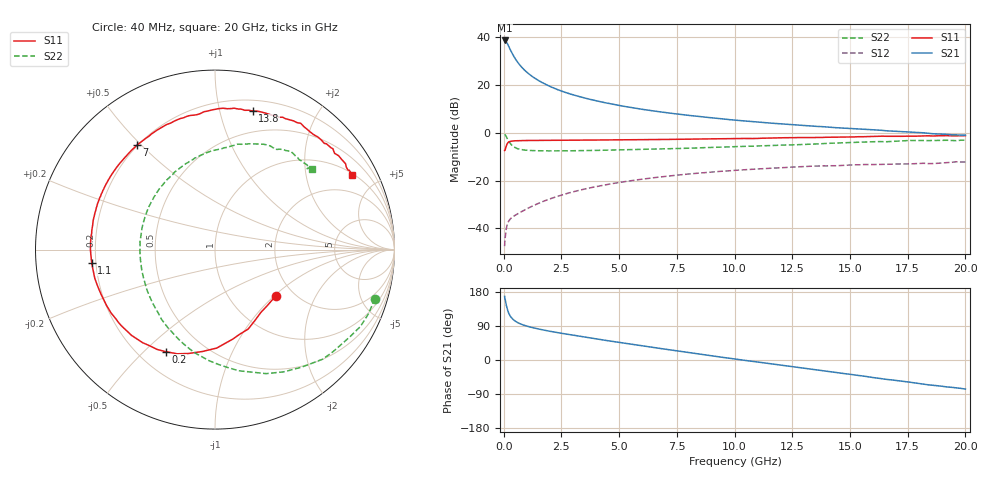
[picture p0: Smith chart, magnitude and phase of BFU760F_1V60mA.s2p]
! Filename:  P:\Prog\Test\Noise\ATS_data\Testdata_Net\Split files Spar\BFU760F_2W_C1_1V_5mA_60mA_Bias9_D.s2p
! Date/Time: Mon 06/Feb/2012 15:06:24
! BFU760_2W_C1_1V_5mA_60mA_Bias9_R.s2p
! MDIF S-parameter v. bias file
! BFU760_2W_C1_1V_5mA_60mA
! Date/time Fri Mar 18 10:56:44 2011
! VAR V_out= 1.0003
! VAR I_out= 60.0200
! VAR V_in= 0.8205
! VAR I_in= 0.2130
! Device data file deembeded for feedlines and parallel
! Original file: \Split files Spar\BFU760_2W_C1_1V_5mA_60mA_Bias9_R.s2p
! Feed-files: PR003V01_101208_Feed1.s2p, PR003V01_101208_Feed2.s2p
! Parallel-file: PR003V01_101208_Par.s2p
# MHz S MA R 50
!  Freq-MHz  S11-mag  S11-arg  S21-mag  S21-arg  S12-mag  S12-arg  S22-mag  S22-arg
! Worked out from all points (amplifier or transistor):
!   167 points, 40 MHz to 20 GHz, reference 50 ohm
!   highest |S21| = 38.7 dB at 40 MHz (marker M1)
!   |S21| within 3 dB of that: start of sweep to 241.6 MHz
!   unconditionally stable (mu >= 1): 2.694 GHz to 15.28 GHz
!   at 550 MHz: K = 0.55, MSG = 32.3 dB, |S12| = -34.3 dB
!   at 4.2 GHz: K = 1.04, MAG = 16.4 dB, |S12| = -22.2 dB
!   at 20 GHz: K = 0.96, MSG = 5.6 dB, |S12| = -12.3 dB
!   S11 on the Smith chart (normalised r, x): 40 MHz: 1.63, -1.02; 200 MHz: 0.31, -0.58; 1.1 GHz: 0.18, -0.05; 7 GHz: 0.20, +0.48; 13.8 GHz: 0.30, +1.26; 20 GHz: 1.06, +3.65
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40  0.4258 -37.1  86.21 167.8  0.004202 78.3  0.9318 -17.1
50  0.4273 -47.5  84.01 162.9  0.005292 70.9  0.9271 -22.6
60  0.4336 -54.0  79.17 160.6  0.005886 71.9  0.9167 -27.8
80  0.48 -67.4  82.28 154.5  0.007572 68.0  0.8807 -36.7
120  0.5486 -89.0  78.46 142.8  0.01019 60.3  0.813 -53.8
180  0.6175 -109.9  71.24 129.7  0.01293 52.3  0.7128 -73.3
200  0.6312 -115.7  67.27 126.2  0.01359 50.4  0.6879 -78.9
260  0.6569 -127.9  58.51 118.2  0.01508 46.7  0.6196 -93.1
300  0.6669 -134.3  53.08 114.3  0.01586 45.2  0.5869 -100.8
380  0.6739 -143.4  45.04 108.6  0.0171 43.6  0.5327 -113.6
480  0.6792 -151.6  37.07 103.3  0.01844 43.5  0.4952 -125.4
750  0.6864 -164.5  24.64 94.7  0.02198 46.2  0.4463 -145.4
1100  0.6906 -174.0  17.02 87.8  0.02693 50.2  0.4271 -159.8
2000  0.6933 172.2  9.4 75.8  0.0411 54.0  0.4186 -179.1
3400  0.7026 157.8  5.532 61.6  0.06442 51.0  0.424 163.8
6800  0.7241 128.4  2.738 30.3  0.1189 32.4  0.4586 132.5
7000  0.7266 126.8  2.656 28.6  0.1218 31.2  0.4623 130.8
10200  0.7592 101.8  1.811 1.1  0.1651 9.9  0.5147 105.4
13400  0.7937 77.9  1.379 -24.9  0.2 -12.6  0.5797 82.0
13800  0.7995 74.8  1.346 -28.2  0.2027 -15.5  0.592 79.2
16800  0.8445 52.6  1.084 -52.5  0.2197 -34.9  0.6577 58.0
20000  0.8709 28.5  0.8908 -76.7  0.2438 -56.4  0.7022 39.8
